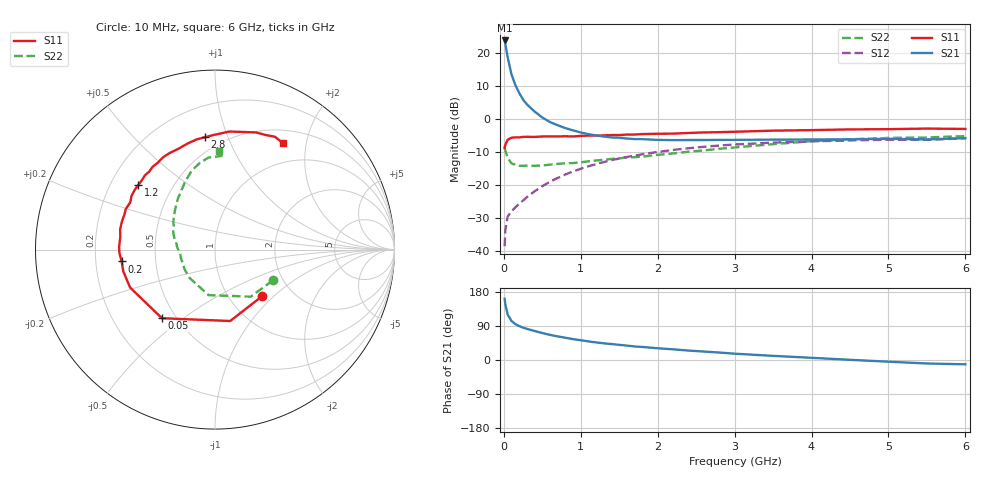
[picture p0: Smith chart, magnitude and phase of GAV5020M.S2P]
! Infineon Technologies  Discrete & RF Semiconductors
! BF775
! Si NPN RF Bipolar Junction Transistor in SOT23
! VCE = 0.5 V  IC = 20 mA
! Common Emitter S-Parameters:  May  1996
# GHz  S  MA  R  50
!  f  S11  S21  S12  S22
! GHz  MAG  ANG  MAG  ANG  MAG  ANG  MAG  ANG
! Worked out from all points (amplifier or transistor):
!   36 points, 10 MHz to 6 GHz, reference 50 ohm
!   highest |S21| = 23.7 dB at 10 MHz (marker M1)
!   |S21| within 3 dB of that: start of sweep to 34 MHz
!   unconditionally stable (mu >= 1): start of sweep to end of sweep
!   at 250 MHz: K = 3.13, MAG = 7.4 dB, |S12| = -24.7 dB
!   at 1.4 GHz: K = 2.75, MAG = -3.8 dB, |S12| = -12.5 dB
!   at 6 GHz: K = 1.19, MAG = -2.6 dB, |S12| = -5.9 dB
!   S11 on the Smith chart (normalised r, x): 10 MHz: 1.41, -0.85; 50 MHz: 0.42, -0.42; 200 MHz: 0.31, -0.06; 1.2 GHz: 0.32, +0.33; 2.8 GHz: 0.40, +0.83; 6 GHz: 0.68, +1.60
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0.01  0.369 -44.8  15.29 161.5  0.0119 67.3  0.3654 -28.0
0.02  0.4067 -78.0  13.47 146.1  0.0211 59.5  0.3291 -52.8
0.05  0.4833 -127.7  8.425 119.8  0.0334 42.3  0.2562 -98.1
0.1  0.5181 -155.9  4.672 102.8  0.0402 40.0  0.2121 -132.2
0.15  0.5251 -166.7  3.23 94.7  0.046 42.8  0.2015 -148.1
0.2  0.5244 -172.8  2.459 89.5  0.0521 47.4  0.1947 -156.0
0.25  0.5329 -178.0  1.953 85.3  0.0583 50.5  0.1949 -162.2
0.3  0.5345 178.7  1.653 82.2  0.0656 53.7  0.1959 -166.2
0.4  0.5326 172.2  1.288 76.5  0.0804 56.8  0.195 -171.4
0.5  0.5406 168.0  1.048 71.2  0.096 58.9  0.1972 -175.8
0.6  0.5416 163.2  0.893 66.3  0.1122 59.4  0.2032 -179.2
0.7  0.5414 158.6  0.8 62.3  0.1277 59.7  0.2084 178.0
0.9  0.5404 150.8  0.669 55.1  0.1602 58.4  0.2146 172.3
1.1  0.5578 143.2  0.587 49.0  0.1917 56.1  0.2277 167.4
1.2  0.5582 140.0  0.56 46.4  0.2072 54.8  0.2346 164.5
1.7  0.5791 123.4  0.494 35.7  0.2779 46.8  0.2633 151.2
2.2  0.5975 109.9  0.477 28.2  0.3388 38.1  0.2999 139.2
2.8  0.6289 95.0  0.48 19.7  0.3949 28.0  0.3522 125.8
3.5  0.6626 83.1  0.485 10.9  0.437 17.0  0.414 113.6
4.5  0.6917 70.7  0.49 0.5  0.4719 4.3  0.4903 99.9
5.5  0.7119 62.0  0.488 -9.2  0.4807 -6.8  0.5231 86.0
6  0.7033 57.6  0.511 -11.4  0.5079 -10.2  0.5475 87.9
